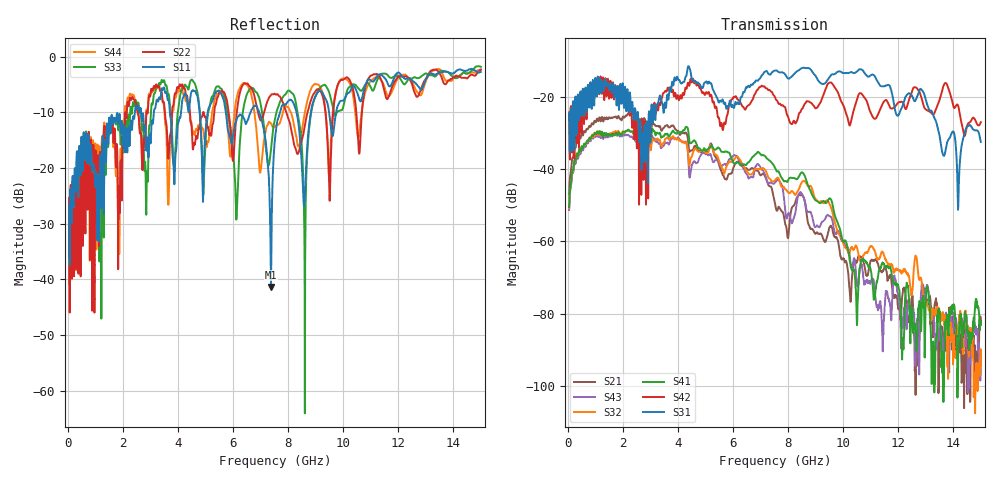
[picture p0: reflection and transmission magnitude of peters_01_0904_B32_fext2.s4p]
# MHZ S RI R 50.00
! FREQ  S11  S12  S13  S14
!  S21  S22  S23  S24
!  S31  S32  S33  S34
!  S41  S42  S43  S44
!  REAL  IMAG  REAL  IMAG  REAL  IMAG  REAL  IMAG
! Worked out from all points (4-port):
!   1496 points, 50 MHz to 15 GHz, reference 50 ohm
!   strongest paths, dB at 50 MHz, 3.79 GHz, 7.53 GHz, 11.27 GHz, 15 GHz:
!     S31: -24.6, -15.9, -12.9, -16.1, -32.5
!     S42: -24.4, -18.4, -20.3, -24.9, -27.1
!     S41: -50.4, -29.7, -39.7, -69.5, -83.1
!     S32: -50.8, -31.3, -43.1, -64.9, -94.5
!     S43: -51.3, -31.6, -43.7, -78.4, -91.0
!     S21: -46.9, -28.1, -49.8, -66.2, -82.8
!   lowest |S11| = -41.3 dB at 7.38 GHz (marker M1), VSWR 1.02, Z = 50.8 - j0.207 ohm
!   |S11| at or under -10 dB: start of sweep to 2.437 GHz; 5.741 GHz to 6.642 GHz (900.2 MHz wide, 14.5 % of centre); 6.953 GHz to 7.707 GHz (754.1 MHz wide, 10.3 % of centre)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
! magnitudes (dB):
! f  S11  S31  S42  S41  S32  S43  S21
! 50 MHz  -26.8  -24.6  -24.4  -50.4  -50.8  -51.3  -46.9
! 2.24 GHz  -16.1  -19.6  -24.5  -29.5  -29.4  -30.9  -24.9
! 5.45 GHz  -6.1  -20.9  -25.7  -34.1  -36.8  -37.6  -37.7
! 7.38 GHz  -41.3  -13.8  -18.6  -38.0  -43.1  -43.8  -44.9
! 7.8 GHz  -8.7  -13.3  -22.3  -42.8  -44.9  -45.3  -51.9
! 10.49 GHz  -6.2  -13.2  -21.0  -81.6  -61.5  -70.6  -65.7
! 15 GHz  -2.8  -32.5  -27.1  -83.1  -94.5  -91.0  -82.8
